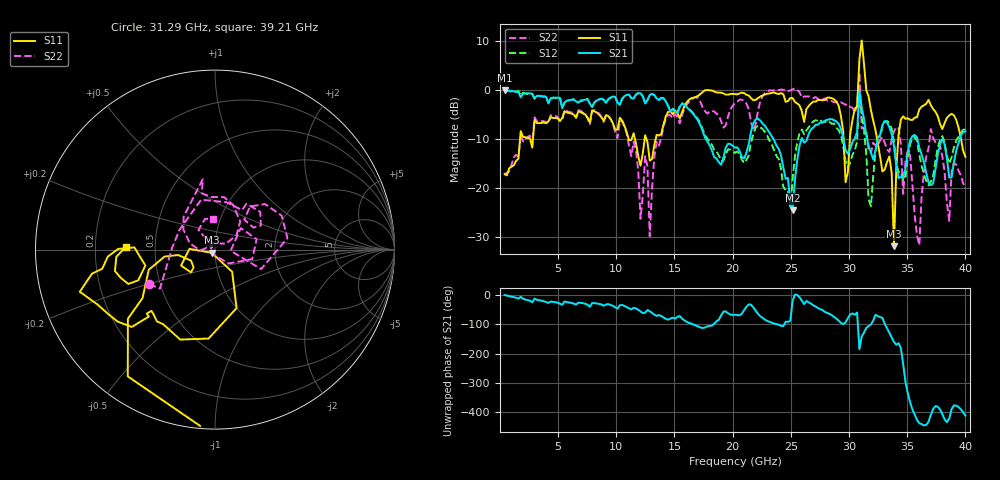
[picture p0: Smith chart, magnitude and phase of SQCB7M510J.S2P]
! Network Analyzer HP8722ES.07.66: Jul 25, 2000 Serial No. US39175408
! 27 Oct 2004  11:09:12
! Frequency  S11  S21  S12  S22
# HZ  S  DB R  50
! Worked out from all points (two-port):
!   201 points, 400 MHz to 40 GHz, reference 50 ohm
!   highest |S21| = -0.12 dB at 400 MHz (marker M1); lowest = -24.6 dB at 25.15 GHz (marker M2)
!   |S21| within 3 dB of the highest: start of sweep to 5.297 GHz; 8.008 GHz to 14.41 GHz (6.399 GHz wide, 57.1 % of centre)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
!   lowest |S11| = -31.9 dB at 33.86 GHz (marker M3), VSWR 1.05, Z = 48.2 - j1.73 ohm
!   |S11| at or under -10 dB: start of sweep to 1.73 GHz; 11.6 GHz to 12.44 GHz (834.6 MHz wide, 6.94 % of centre); 32.41 GHz to 34.23 GHz (1.829 GHz wide, 5.49 % of centre)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
!   |S22| runs from -31.7 to 3.5 dB; largest |S21 - S12| = 0.2
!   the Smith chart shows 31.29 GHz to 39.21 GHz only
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4e8  -17.16 -94.3  -0.12 0.5  -0.05 1.4  -17.40 -91.3
7.132e9  -4.81 -107.3  -2.08 -27.5  -2.17 -28.5  -4.67 -126.0
1.1488e10  -8.84 -87.4  -1.78 -43.1  -1.77 -43.5  -10.60 -127.2
1.2082e10  -15.47 -62.7  -0.70 -55.4  -0.71 -56.3  -26.28 -156.5
1.2478e10  -9.25 -43.2  -2.78 -59.9  -2.81 -60.2  -13.53 -57.7
1.2874e10  -14.42 -51.2  -1.05 -55.0  -1.06 -55.8  -29.84 -99.1
1.3666e10  -9.30 -14.1  -2.09 -68.4  -1.95 -68.4  -11.37 -11.9
2.02e10  -0.86 -3.5  -11.80 -67.1  -12.84 -72.2  -2.70 -14.5
2.515e10  -1.68 -86.4  -24.57 -19.6  -18.17 3.7  0.09 -24.3
2.6932e10  -2.40 131.8  -7.69 -34.8  -6.46 -46.0  -1.68 -29.9
2.9704e10  -18.85 -25.7  -12.31 -93.3  -14.47 -106.2  -3.05 -57.9
3.0496e10  -3.87 84.8  -9.94 -67.0  -12.31 -68.3  -4.61 -90.1
3.0694e10  -3.40 70.3  -8.55 -59.5  -10.54 -60.1  -3.32 -112.6
3.0892e10  6.22 19.5  -0.19 175.1  -0.52 168.9  3.53 30.7
3.109e10  10.07 -76.5  -3.59 -141.5  -5.20 -150.3  -7.86 163.9
3.1486e10  -0.12 -94.8  -9.28 -111.9  -13.24 -140.9  -8.50 -144.7
3.1882e10  -4.15 -141.5  -12.78 -100.6  -23.71 -49.8  -12.90 150.7
3.3466e10  -13.59 -154.7  -7.60 -128.6  -6.77 -108.3  -12.65 45.6
3.3862e10  -31.86 -135.4  -11.44 -160.0  -10.48 -145.9  -8.47 42.3
3.4654e10  -5.39 -111.1  -17.87 124.2  -18.42 146.3  -21.19 -4.3
3.703e10  -3.12 -168.9  -19.43 -49.9  -18.72 -30.1  -8.00 99.8
4e10  -13.65 -168.1  -8.46 -52.3  -8.07 -55.8  -20.01 83.9
